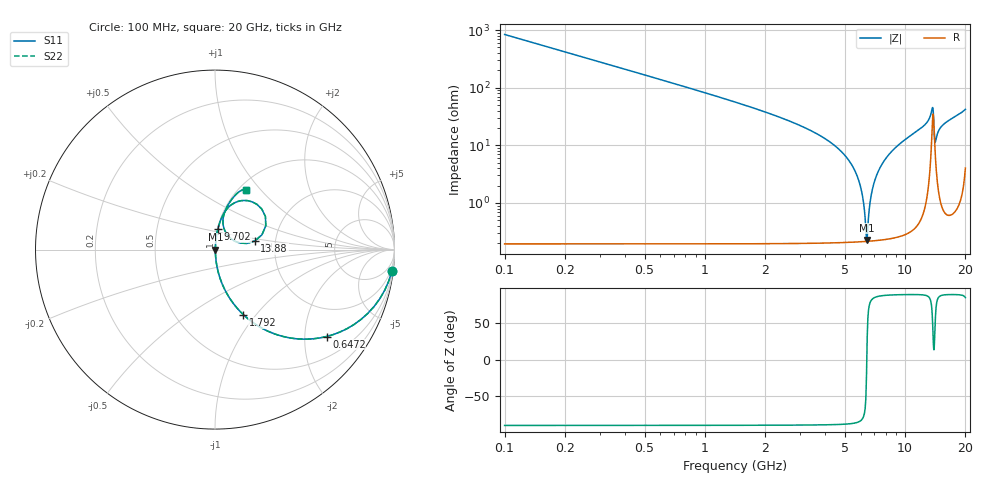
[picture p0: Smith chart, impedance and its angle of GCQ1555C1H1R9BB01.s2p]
!Murata Part Number: GCQ1555C1H1R9BB01
!These Parameters are Measured in Series Mode Connection
!Data Generated on Jan 08, 2026
!  o--ll--o
!Port1  Port2
!  o------o
!Operation Temp=25[degC], DC Bias Voltage=0[V]
!Freq. Start=100[MHz] Stop=20[GHz] 401[Steps]
# Hz S RI R 50
!Freq.(Hz) S11(Real) S11(Imag) S21(Real) S21(Imag) S12(Real) S12(Imag) S22(Real) S22(Imag)
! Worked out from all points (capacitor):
!   401 points, 100 MHz to 20 GHz, reference 50 ohm
!   read as one part in series: C = 1.9 pF near 199.5 MHz
!   lowest |Z| = 228 mohm at 6.418 GHz (marker M1)
!   series resonance near 6.436 GHz, so ESL is about 320 pH
!   S11 on the Smith chart (normalised r, x): 100 MHz: 1, -17; 647.2 MHz: 1.00, -2.56; 1.792 GHz: 1.00, -0.86; 9.702 GHz: 1.01, +0.23; 13.88 GHz: 1.56, +0.16; 20 GHz: 1.08, +0.84
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1e8  0.9859 -0.1177  0.0141 0.1177  0.0141 0.1177  0.9859 -0.1177
3.4875e8  0.8513 -0.3554  0.1487 0.3554  0.1487 0.3554  0.8513 -0.3554
6.4725e8  0.6213 -0.4843  0.3787 0.4843  0.3787 0.4843  0.6213 -0.4843
1.14475e9  0.3349 -0.4706  0.6651 0.4706  0.6651 0.4706  0.3349 -0.4706
1.7915e9  0.1583 -0.3628  0.8417 0.3628  0.8417 0.3628  0.1583 -0.3628
3.43325e9  0.0317 -0.1695  0.9683 0.1695  0.9683 0.1695  0.0317 -0.1695
5.62225e9  0.00337 -0.0356  0.9966 0.0356  0.9966 0.0356  0.00337 -0.0356
6.07e9  0.00236 -0.0154  0.9976 0.0154  0.9976 0.0154  0.00236 -0.0154
6.41825e9  0.00215 -0.000745  0.9978 0.000745  0.9978 0.000745  0.00215 -0.000745
6.51775e9  0.00217 0.00332  0.9978 -0.00332  0.9978 -0.00332  0.00217 0.00332
6.7665e9  0.00236 0.0132  0.9976 -0.0132  0.9976 -0.0132  0.00236 0.0132
7.11475e9  0.00293 0.0266  0.9971 -0.0266  0.9971 -0.0266  0.00293 0.0266
7.71175e9  0.00463 0.0483  0.9954 -0.0483  0.9954 -0.0483  0.00463 0.0483
9.70175e9  0.0159 0.1139  0.9841 -0.1139  0.9841 -0.1139  0.0159 0.1139
1.005e10  0.0187 0.1247  0.9813 -0.1247  0.9813 -0.1247  0.0187 0.1247
1.338325e10  0.1311 0.2693  0.8689 -0.2693  0.8689 -0.2693  0.1311 0.2693
1.368175e10  0.261 0.2256  0.739 -0.2256  0.739 -0.2256  0.261 0.2256
1.388075e10  0.2223 0.0482  0.7777 -0.0482  0.7777 -0.0482  0.2223 0.0482
1.41295e10  0.0747 0.0744  0.9253 -0.0744  0.9253 -0.0744  0.0747 0.0744
1.497525e10  0.0478 0.188  0.9522 -0.188  0.9522 -0.188  0.0478 0.188
1.67165e10  0.0763 0.2548  0.9237 -0.2548  0.9237 -0.2548  0.0763 0.2548
2e10  0.1734 0.3336  0.8266 -0.3336  0.8266 -0.3336  0.1734 0.3336
